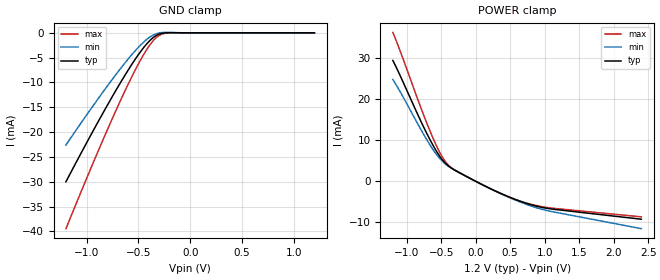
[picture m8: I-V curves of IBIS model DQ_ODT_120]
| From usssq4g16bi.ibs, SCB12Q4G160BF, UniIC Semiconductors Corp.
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|   Model DQ_ODT_120
[Model] DQ_ODT_120
Model_type Input
Polarity   Non-Inverting
Enable   Active-High
Vinl =  8.300E-01
Vinh =  9.700E-01
C_comp   8.303E-13   8.275E-13   8.387E-13
C_comp_power_clamp   2.806E-13   2.784E-13   2.809E-13
C_comp_gnd_clamp   5.519E-13   5.466E-13   5.581E-13
[Model Spec]
Vinh   9.700E-01   9.250E-01   1.015E+00
Vinl   8.300E-01   7.850E-01   8.750E-01
[Temperature Range]   45.000   95.000   -40.000
[Voltage Range]   1.200E+00   1.140E+00   1.260E+00
[C Comp Corner]
C_comp_power_clamp   2.784E-13   2.806E-13   2.809E-13
C_comp_gnd_clamp   5.519E-13   5.581E-13   5.466E-13
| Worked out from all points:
|   GND clamp passes 1 mA (typ) near -0.36 V on its own axis
|   POWER clamp passes 1 mA (typ) near -0.11 V on its own axis
[GND_clamp]
|Voltage   I(typ)   I(min)   I(max)
-1.2V     -30mA      -22.6mA    -39.46mA
-875mV    -17.38mA   -12.86mA   -23.15mA
-750mV    -12.76mA   -9.302mA   -17.17mA
-625mV    -8.371mA   -5.935mA   -11.48mA
-525mV    -5.133mA   -3.476mA   -7.242mA
-450mV    -2.983mA   -1.877mA   -4.387mA
-375mV    -1.263mA   -657.6uA   -2.026mA
-325mV    -500.7uA   -167.9uA   -904.9uA
-275mV    -110uA     47.1uA     -266.8uA
-200mV    26.77uA    83.14uA    363.2nA
1.2V      0A         0A         0A
[POWER_clamp]
|Voltage   I(typ)   I(min)   I(max)
-1.2V     29.47mA    24.83mA    36.31mA
-1.075V   25.07mA    21.28mA    30.9mA
-775mV    13.98mA    12.07mA    17.11mA
-625mV    8.999mA    7.909mA    10.81mA
-550mV    6.847mA    6.174mA    8.033mA
-475mV    5.079mA    4.774mA    5.694mA
-425mV    4.182mA    4.043mA    4.493mA
-350mV    3.206mA    3.178mA    3.287mA
300mV     -2.482mA   -2.509mA   -2.498mA
800mV     -5.707mA   -6.008mA   -5.609mA
1.125V    -6.812mA   -7.458mA   -6.579mA
2.4V      -9.248mA   -11.55mA   -8.674mA
